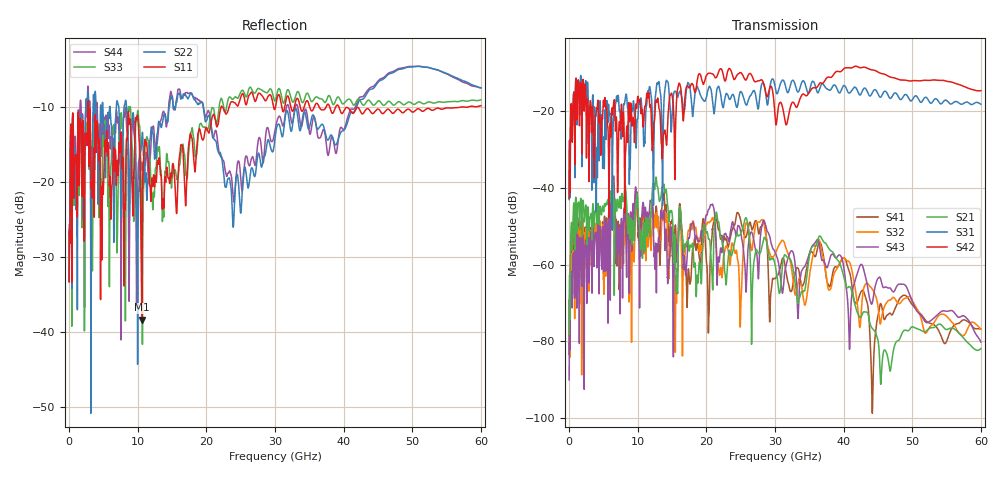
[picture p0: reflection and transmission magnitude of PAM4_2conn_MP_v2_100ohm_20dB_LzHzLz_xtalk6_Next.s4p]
! Info: Touchstone file created by Circ.  Input file=FAB50GbE_2conn_Midplane_Examax_Topo2_v2_100ohm_20dB_LzHzLz.circ
# Hz S RI R 50
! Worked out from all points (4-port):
!   6000 points, 10 MHz to 60 GHz, reference 50 ohm
!   strongest paths, dB at 10 MHz, 15.01 GHz, 30.01 GHz, 45.01 GHz, 60 GHz:
!     S42: -42.6, -15.7, -21.2, -9.7, -14.6
!     S31: -43.0, -21.6, -13.4, -15.4, -18.1
!     S21: -78.3, -46.4, -59.9, -79.8, -82.0
!     S43: -90.1, -54.2, -56.8, -63.6, -80.2
!     S32: -78.7, -52.8, -57.3, -70.9, -76.9
!     S41: -83.5, -48.5, -63.7, -73.5, -76.9
!   lowest |S11| = -38.4 dB at 10.59 GHz (marker M1), VSWR 1.02, Z = 48.8 + j0.296 ohm
!   |S11| at or under -10 dB: start of sweep to 2.748 GHz; 2.836 GHz to 22.12 GHz (19.29 GHz wide, 155 % of centre); 39.33 GHz to 56.93 GHz (17.6 GHz wide, 36.6 % of centre)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
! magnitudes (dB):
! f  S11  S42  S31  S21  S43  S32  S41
! 10 MHz  -33.3  -42.6  -43.0  -78.3  -90.1  -78.7  -83.5
! 1.18 GHz  -24.7  -20.2  -22.0  -49.5  -56.4  -55.2  -52.8
! 10.59 GHz  -38.4  -19.4  -19.3  -52.9  -49.1  -48.1  -49.2
! 12.51 GHz  -19.9  -20.8  -17.3  -40.0  -61.2  -49.9  -49.3
! 18.62 GHz  -15.4  -12.6  -13.5  -63.7  -52.8  -53.1  -54.9
! 25.75 GHz  -9.7  -11.8  -18.2  -47.8  -66.3  -49.2  -52.9
! 60 GHz  -9.8  -14.6  -18.1  -82.0  -80.2  -76.9  -76.9
